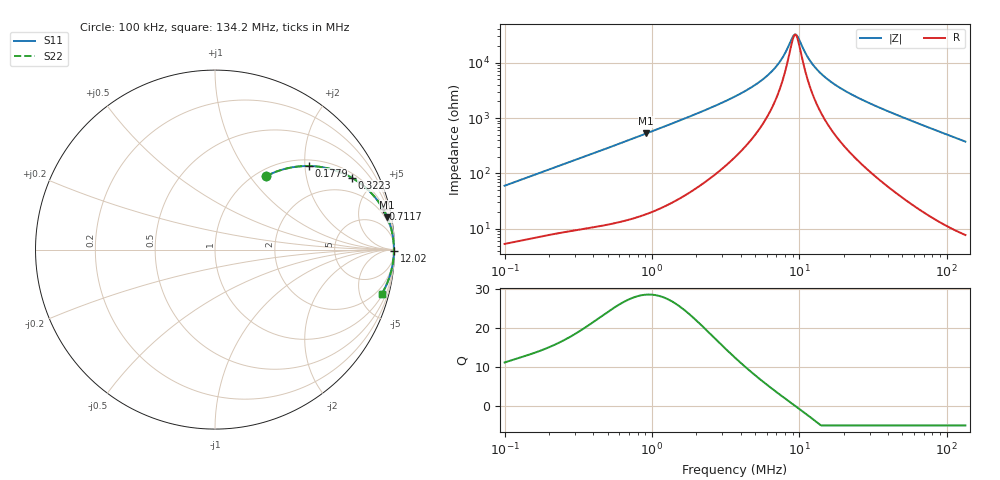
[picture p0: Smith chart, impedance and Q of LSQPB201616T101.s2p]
! LSQPB201616T101  S-PARAMETER MODEL  ( General Type )
! Model Generated by TAIYO YUDEN Corporation (http://www.ty-top.com)
! Version 2.0
! TAIYO YUDEN Control No. 100810NC14SB-FKC
! Copyright(c) 2008 TAIYO YUDEN CO.,LTD. All Rights Reserved.
! Product Description (link to TY-COMPAS)
! https://ds.yuden.co.jp/TYCOMPAS/or/detail?pn=LSQPB201616T101K&u=M
! Products Name : Inductors
! Characteristics :
!  Inductance : 100 uH , SRF(min) : 7.0 MHz , DC Resistance(max) : 4.42 Ohm
!  Rated Current : Saturation :140 mA , Temp Rise : 170 mA (40 degC)
!  Case Size : 2.0 x 1.6 / 0.079 x 0.063 [mm/inch] , Thickness : 1.6 / 0.063 [mm/inch]
!  (Conditions: Temperature = 25 degC , DC Bias Current/Voltage = 0A / 0V)
! External Node Assignments :
!  1  o---GGG---o  2
! GND o---------o GND
! Frequency Range : 0.1MHz  -  134.160692MHz  [ 402 STEP ]
# MHz S RI R 50
! Freq[MHz].  S11 Real  S11 Imag  S21 Real  S21 Imag  S12 Real  S12 Imag  S22 Real  S22 Imag
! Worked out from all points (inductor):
!   401 points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, 100 kHz to 134.2 MHz, reference 50 ohm
!   read as one part in series: L = 94.4 uH near 103.7 kHz
!   highest Q = 28.6 at 915.7 kHz (marker M1), where L = 91.6 uH
!   self-resonance near 9.341 MHz
!   S11 on the Smith chart (normalised r, x): 100 kHz: 1.11, +1.19; 177.9 kHz: 1.15, +2.09; 322.3 kHz: 1.19, +3.72; 711.7 kHz: 1.30, +8.17; 12.02 MHz: open; 134.2 MHz: 1.15, -7.52
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0.1  0.2818 0.4073  0.7182 -0.4073  0.7182 -0.4073  0.2818 0.4073
0.177914  0.5215 0.4658  0.4785 -0.4658  0.4785 -0.4658  0.5215 0.4658
0.322284  0.765 0.3987  0.235 -0.3987  0.235 -0.3987  0.765 0.3987
0.334101  0.777 0.3915  0.223 -0.3915  0.223 -0.3915  0.777 0.3915
0.711669  0.9362 0.2269  0.0638 -0.2269  0.0638 -0.2269  0.9362 0.2269
0.915682  0.9594 0.1807  0.0406 -0.1807  0.0406 -0.1807  0.9594 0.1807
1.116232  0.9715 0.1497  0.0285 -0.1497  0.0285 -0.1497  0.9715 0.1497
2.293596  0.9913 0.0711  0.00872 -0.0711  0.00872 -0.0711  0.9913 0.0711
3.729338  0.9952 0.0394  0.00482 -0.0394  0.00482 -0.0394  0.9952 0.0394
5.156735  0.9963 0.0236  0.00372 -0.0236  0.00372 -0.0236  0.9963 0.0236
6.516624  0.9967 0.0139  0.00331 -0.0139  0.00331 -0.0139  0.9967 0.0139
7.52619  0.9968 0.00831  0.00317 -0.00831  0.00317 -0.00831  0.9968 0.00831
9.010851  0.9969 0.00155  0.00309 -0.00155  0.00309 -0.00155  0.9969 0.00155
9.341227  0.9969 0.000208  0.00308 -0.000208  0.00308 -0.000208  0.9969 0.000208
9.859641  0.9969 -0.0018  0.00308 0.0018  0.00308 0.0018  0.9969 -0.0018
10.98438  0.9969 -0.00584  0.00311 0.00584  0.00311 0.00584  0.9969 -0.00584
12.01907  0.9968 -0.00926  0.00316 0.00926  0.00316 0.00926  0.9968 -0.00926
12.23742  0.9968 -0.00995  0.00318 0.00995  0.00318 0.00995  0.9968 -0.00995
14.65145  0.9966 -0.0171  0.00337 0.0171  0.00337 0.0171  0.9966 -0.0171
18.85157  0.9961 -0.028  0.00388 0.028  0.00388 0.028  0.9961 -0.028
40.88529  0.9909 -0.0762  0.00912 0.0762  0.00912 0.0762  0.9909 -0.0762
134.1607  0.9296 -0.2458  0.0704 0.2458  0.0704 0.2458  0.9296 -0.2458
